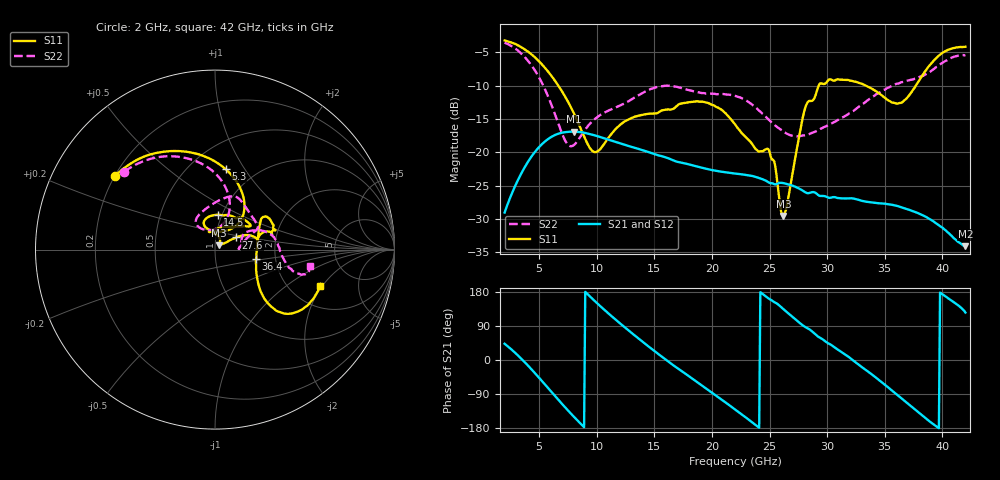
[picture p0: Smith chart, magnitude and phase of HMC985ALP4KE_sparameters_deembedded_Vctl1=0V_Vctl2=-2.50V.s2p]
!s2p File: Measurements: S11, S21, S12, S22
# GHz S dB R 50.0
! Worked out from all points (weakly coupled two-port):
!   401 points, 2 GHz to 42 GHz, reference 50 ohm
!   highest |S21| = -16.89 dB at 8 GHz (marker M1); lowest = -34.1 dB at 42 GHz (marker M2)
!   lowest |S11| = -29.5 dB at 26.2 GHz (marker M3), VSWR 1.07, Z = 52.3 + j2.52 ohm
!   |S11| at or under -10 dB: 6.669 GHz to 29.26 GHz (22.59 GHz wide, 126 % of centre); 33.38 GHz to 37.7 GHz (4.322 GHz wide, 12.2 % of centre)
!   |S22| runs from -19.1 to -3.5 dB; largest |S21 - S12| = 0.00054
!   S11 on the Smith chart (normalised r, x): 2 GHz: 0.20, +0.32; 5.3 GHz: 0.73, +0.83; 14.5 GHz: 0.95, +0.39; 27.6 GHz: 1.25, +0.17; 36.4 GHz: 1.58, -0.18; 42 GHz: 2.91, -1.90
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2  -3.20 143.5  -29.04 43.0  -29.03 42.9  -3.53 139.2
3.5  -4.27 116.7  -23.00 1.8  -23.02 1.8  -5.26 109.6
5.3  -6.91 82.4  -18.68 -57.6  -18.70 -57.6  -9.78 77.3
7.2  -11.47 52.7  -16.98 -123.2  -17.00 -123.2  -18.03 80.4
8  -14.08 48.4  -16.89 -149.3  -16.88 -149.3  -18.92 106.8
8.7  -16.83 52.5  -17.00 -171.2  -17.00 -171.2  -17.33 122.2
10  -19.92 89.8  -17.54 150.6  -17.53 150.6  -14.75 125.5
14.5  -14.21 85.7  -19.96 35.5  -19.93 35.6  -10.64 79.0
15.4  -13.96 73.5  -20.48 14.5  -20.49 14.5  -10.12 72.3
19.3  -12.43 34.0  -22.38 -70.8  -22.38 -70.8  -11.10 43.2
22  -15.78 52.3  -23.18 -130.3  -23.20 -130.4  -11.52 26.4
25  -19.95 98.9  -24.59 160.8  -24.56 160.9  -15.23 16.9
26.2  -29.53 46.2  -24.62 134.3  -24.65 134.3  -16.88 7.1
27.6  -17.33 29.9  -25.46 98.2  -25.47 98.1  -17.52 1.9
28.1  -13.28 21.0  -25.99 87.1  -26.04 87.0  -17.43 3.5
28.7  -12.26 13.0  -25.97 75.3  -25.98 75.2  -17.07 7.5
31  -9.05 23.3  -26.87 26.0  -26.85 25.9  -15.06 27.6
33.3  -9.93 34.2  -27.37 -25.0  -27.36 -25.0  -12.49 26.6
35.4  -12.27 12.0  -27.80 -75.0  -27.79 -74.9  -10.22 17.9
36.4  -12.58 -13.2  -28.21 -100.1  -28.25 -100.2  -9.49 12.1
39.5  -5.82 -43.4  -30.70 -175.5  -30.65 -175.7  -7.16 -14.3
42  -4.15 -19.0  -34.08 125.2  -34.09 125.0  -5.39 -10.0
